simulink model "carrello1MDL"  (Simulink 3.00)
settings: Solver=ode45  SolverMode=SingleTasking  StartTime=0.0  StopTime=10.0  RelTol=1e-6  AbsTol=1e-7
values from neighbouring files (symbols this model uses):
  A_dis = 1*10*cm    (= 0.1)    [carrello2.M]    (also in carrello1.M)
  b1 = 2*1500*N/(m/sec)    (= 3000)    [carrello2.M]    (also in carrello3.M; carrello4.M; carrello5.M; carrello6.M)
  b2 = 2*1500*N/(m/sec)    (= 3000)    [carrello2.M]    (also in carrello3.M; carrello4.M; carrello5.M; carrello6.M)
  F = 1    [carrello2.M]    (also in carrello3.M; carrello1.M = 0)
  Freq_dis = 1*5*rad/sec    (= 5)    [carrello2.M]    (also in carrello1.M)
  K = 0.8*1800*N/cm    (= 144000)    [carrello2.M]    (also in carrello3.M; carrello4.M; carrello5.M; carrello6.M)
  Kp = 2*1800*N/cm    (= 360000)    [carrello2.M]    (also in carrello3.M; carrello4.M; carrello5.M; carrello6.M)
  Ma = 3850*Kg    (= 3850)    [carrello2.M]    (also in carrello3.M; carrello4.M; carrello5.M; carrello6.M)
  Mag = Ma*g    (= 37768.5)    [carrello2.M]    (also in carrello3.M = 0; carrello1.M)
  mr = 2*134*Kg+524*Kg    (= 792)    [carrello2.M]    (also in carrello3.M; carrello4.M; carrello5.M; carrello6.M)
  mrg = mr*g    (= 7769.52)    [carrello2.M]    (also in carrello3.M = 0; carrello1.M)
  X_12_0 = -Mag/K    (= -0.26228125)    [carrello2.M]    (also in carrello3.M = 0; carrello4.M = 0; carrello5.M = 0; carrello6.M = 0)
  X_20_0 = -(Mag+mrg)/Kp    (= -0.1264945)    [carrello2.M]    (also in carrello3.M = 0; carrello4.M = 0; carrello5.M = 0; carrello6.M = 0)
libraries: simulink3 x6, cstblocks x2

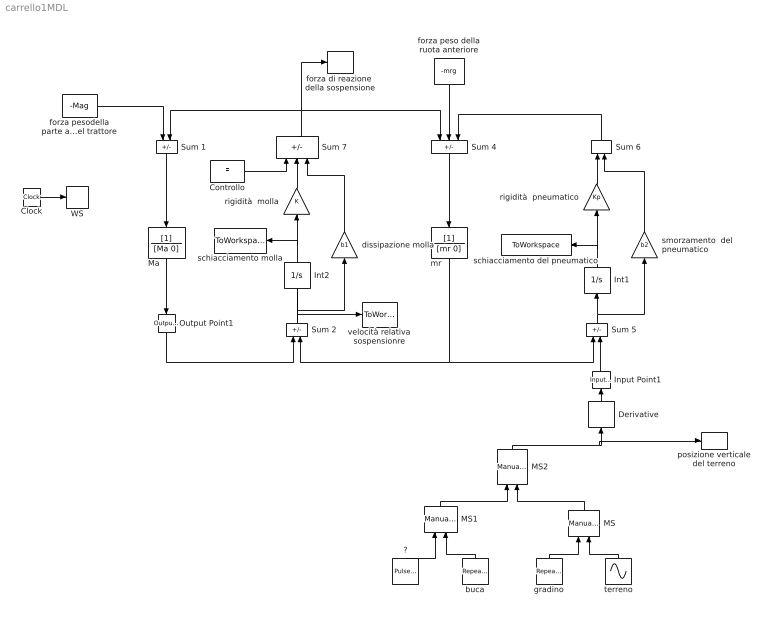
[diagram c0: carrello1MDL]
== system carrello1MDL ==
  "?" : simulink3/Sources/Pulse Generator  Orientation=up  period=1  duty=50  amplitude=0  start=0
  Clock : Clock
  Controllo : Constant  Value=F
  Derivative : Derivative  Orientation=up
  Input Point1 : cstblocks/Input Point  Orientation=up  PerturbationValue=0
  Int1 : Integrator  Orientation=up  ExternalReset=none  InitialConditionSource=internal  InitialCondition=X_20_0  LimitOutput=off  UpperSaturationLimit=inf  LowerSaturationLimit=-inf  ShowSaturationPort=off  ShowStatePort=off  AbsoluteTolerance=auto
  Int2 : Integrator  Orientation=up  ExternalReset=none  InitialConditionSource=internal  InitialCondition=X_12_0  LimitOutput=off  UpperSaturationLimit=inf  LowerSaturationLimit=-inf  ShowSaturationPort=off  ShowStatePort=off  AbsoluteTolerance=auto
  MS : simulink3/Nonlinear/Manual Switch  Orientation=up  sw=1  action=0
  MS1 : simulink3/Nonlinear/Manual Switch  Orientation=up  sw=1  action=0
  MS2 : simulink3/Nonlinear/Manual Switch  Orientation=up  sw=0  action=0
  Ma : TransferFcn  Orientation=down  Numerator=[1]  Denominator=[Ma 0]
  Output Point1 : cstblocks/Output Point  Orientation=down  SigprobeOutputIndex=1
  Sum 1 : Sum  Orientation=down  Inputs=+-  SaturateOnIntegerOverflow=on
  Sum 2 : Sum  Orientation=up  Inputs=+-
  Sum 4 : Sum  Orientation=down  Inputs=++-
  Sum 5 : Sum  Orientation=up  Inputs=+-
  Sum 6 : Sum  Orientation=up  Inputs=++
  Sum 7 : Sum  Orientation=up  Inputs=-++
  WS : ToWorkspace  VariableName=t  SampleTime=-1  SaveFormat=Matrix
  buca : simulink3/Sources/Repeating Sequence  Orientation=up  rep_seq_t=[0 1 1.01 3 3.01 10]  rep_seq_y=[0 0 -0.1 -0.1 0 0]
  dissipazione molla : Gain  Orientation=up  Gain=b1  SaturateOnIntegerOverflow=on
  forza di reazione  della sospensione : ToWorkspace  VariableName=R  SampleTime=-1  SaveFormat=Matrix
  forza peso della ruota anteriore : Constant  Orientation=down  Value=-mrg
  forza pesodella parte anteriore del trattore : Constant  Value=-Mag
  gradino : simulink3/Sources/Repeating Sequence  Orientation=up  rep_seq_t=[0 1 1.01 3 3.01 10]  rep_seq_y=[0 0 0.1 0.1 0 0]
  mr : TransferFcn  Orientation=down  Numerator=[1]  Denominator=[mr 0]
  posizione verticale del terreno : ToWorkspace  VariableName=Xs  SampleTime=-1  SaveFormat=Matrix
  rigidità  molla : Gain  Orientation=up  Gain=K  SaturateOnIntegerOverflow=on
  rigidità  pneumatico : Gain  Orientation=up  Gain=Kp  SaturateOnIntegerOverflow=on
  schiacciamento del pneumatico : ToWorkspace  VariableName=X_20  SampleTime=-1  SaveFormat=Matrix
  schiacciamento molla : ToWorkspace  VariableName=X_12  SampleTime=-1  SaveFormat=Matrix
  smorzamento  del pneumatico : Gain  Orientation=up  Gain=b2  SaturateOnIntegerOverflow=on
  terreno : Sin  Orientation=up  Amplitude=A_dis  Frequency=Freq_dis  Phase=0  SampleTime=0
  velocità relativa sospensionre : ToWorkspace  VariableName=vel_rel  SampleTime=-1  SaveFormat=Matrix
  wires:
  forza pesodella parte anteriore del trattore/1 -> Sum 1/1
  Sum 1/1 -> Ma/1
  forza peso della ruota anteriore/1 -> Sum 4/2
  Sum 4/1 -> mr/1
  mr/1 -> Sum 5/1, Sum 2/2
  Int1/1 -> rigidità  pneumatico/1, schiacciamento del pneumatico/1
  Sum 5/1 -> Int1/1, smorzamento  del pneumatico/1
  rigidità  pneumatico/1 -> Sum 6/1
  smorzamento  del pneumatico/1 -> Sum 6/2
  Clock/1 -> WS/1
  Sum 7/1 -> Sum 1/2, forza di reazione  della sospensione/1, Sum 4/1
  Sum 6/1 -> Sum 4/3
  Sum 2/1 -> velocità relativa sospensionre/1, Int2/1, dissipazione molla/1
  Int2/1 -> rigidità  molla/1, schiacciamento molla/1
  terreno/1 -> MS/2
  gradino/1 -> MS/1
  MS1/1 -> MS2/1
  MS/1 -> MS2/2
  "?"/1 -> MS1/1
  buca/1 -> MS1/2
  MS2/1 -> posizione verticale del terreno/1, Derivative/1
  Derivative/1 -> Input Point1/1
  Input Point1/1 -> Sum 5/2
  Ma/1 -> Output Point1/1
  Output Point1/1 -> Sum 2/1
  dissipazione molla/1 -> Sum 7/3
  rigidità  molla/1 -> Sum 7/2
  Controllo/1 -> Sum 7/1
